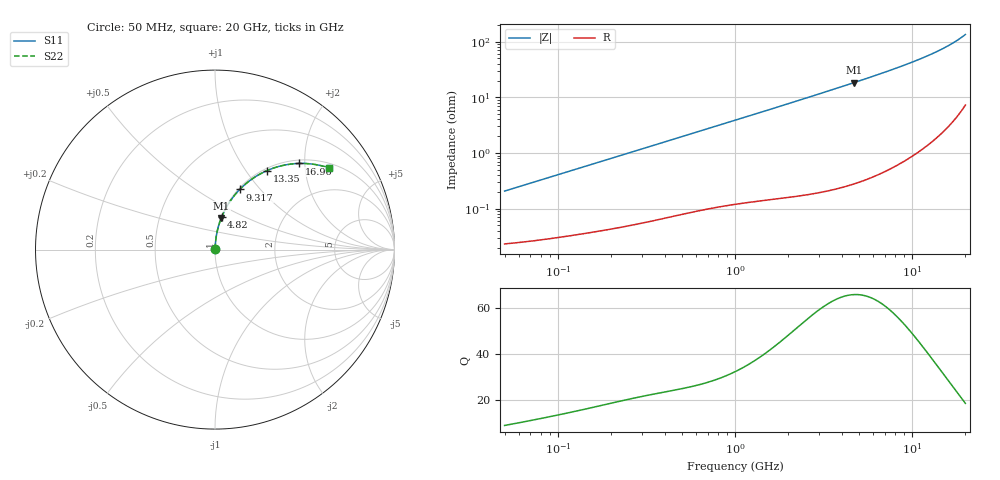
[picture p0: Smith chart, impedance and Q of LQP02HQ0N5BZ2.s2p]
!Murata Part Number: LQP02HQ0N5BZ2
!These Parameters are Measured in Series Mode Connection
!  o--[Z]--o
!Port1  Port2
!  o-------o
!Freq. Start=50[MHz] Stop=20[GHz], 401[Steps]
# Hz S RI R 50
!Freq.(Hz) S11(Real) S11(Imag) S21(Real) S21(Imag) S12(Real) S12(Imag) S22(Real) S22(Imag)
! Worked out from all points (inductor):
!   401 points, 50 MHz to 20 GHz, reference 50 ohm
!   read as one part in series: L = 653 pH near 51.52 MHz
!   highest Q = 65.9 at 4.678 GHz (marker M1), where L = 621 pH
!   S11 on the Smith chart (normalised r, x): 50 MHz: 1.00, +0.00; 4.82 GHz: 1.01, +0.38; 9.317 GHz: 1.02, +0.78; 13.35 GHz: 1.03, +1.26; 16.96 GHz: 1.07, +1.88; 20 GHz: 1.15, +2.68
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5e7  0.000238 0.00206  0.9998 -0.00206  0.9998 -0.00206  0.000238 0.00206
5.152053e7  0.00024 0.00212  0.9998 -0.00212  0.9998 -0.00212  0.00024 0.00212
1.364002e8  0.000382 0.0055  0.9996 -0.0055  0.9996 -0.0055  0.000382 0.0055
3.721004e8  0.000855 0.0147  0.9991 -0.0147  0.9991 -0.0147  0.000855 0.0147
1e9  0.00268 0.0385  0.9973 -0.0385  0.9973 -0.0385  0.00268 0.0385
1.714689e9  0.0058 0.0654  0.9942 -0.0654  0.9942 -0.0654  0.0058 0.0654
2.728004e9  0.0127 0.1035  0.9873 -0.1035  0.9873 -0.1035  0.0127 0.1035
3.626126e9  0.0214 0.137  0.9786 -0.137  0.9786 -0.137  0.0214 0.137
4.677679e9  0.0348 0.1758  0.9652 -0.1758  0.9652 -0.1758  0.0348 0.1758
4.81993e9  0.0369 0.181  0.9631 -0.181  0.9631 -0.181  0.0369 0.181
6.125241e9  0.0591 0.228  0.9409 -0.228  0.9409 -0.228  0.0591 0.228
7.442007e9  0.0872 0.2739  0.9128 -0.2739  0.9128 -0.2739  0.0872 0.2739
9.316812e9  0.1378 0.3352  0.8622 -0.3352  0.8622 -0.3352  0.1378 0.3352
1.034674e10  0.171 0.3661  0.829 -0.3661  0.829 -0.3661  0.171 0.3661
1.131968e10  0.2058 0.393  0.7942 -0.393  0.7942 -0.393  0.2058 0.393
1.238412e10  0.2478 0.4194  0.7522 -0.4194  0.7522 -0.4194  0.2478 0.4194
1.334722e10  0.2893 0.44  0.7107 -0.44  0.7107 -0.44  0.2893 0.44
1.504638e10  0.3697 0.467  0.6303 -0.467  0.6303 -0.467  0.3697 0.467
1.696185e10  0.4694 0.4801  0.5306 -0.4801  0.5306 -0.4801  0.4694 0.4801
1.828096e10  0.5416 0.4765  0.4584 -0.4765  0.4584 -0.4765  0.5416 0.4765
1.940974e10  0.604 0.4645  0.396 -0.4645  0.396 -0.4645  0.604 0.4645
2e10  0.6363 0.4547  0.3637 -0.4547  0.3637 -0.4547  0.6363 0.4547
